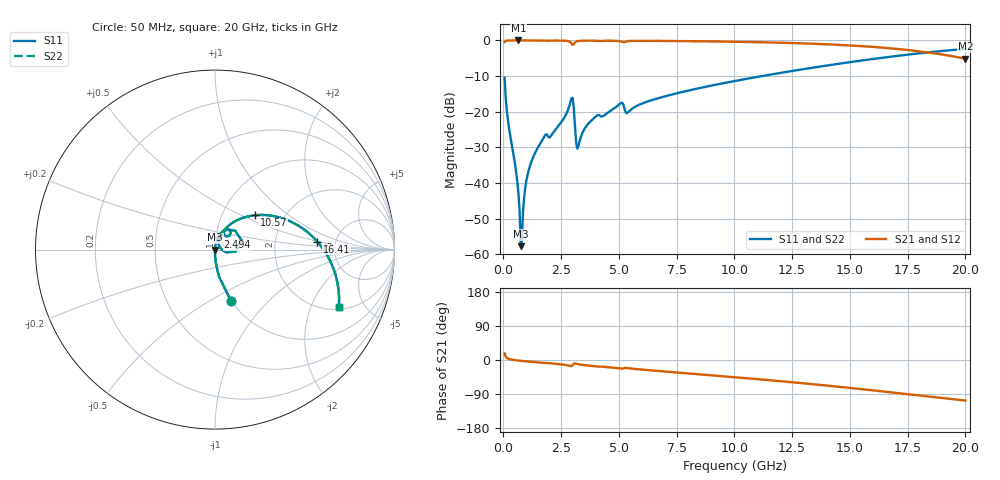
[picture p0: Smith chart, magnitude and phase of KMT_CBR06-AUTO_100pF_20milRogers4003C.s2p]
! Data measured by Modelithics Inc. support@modelithics.com 813-866-6335
! KEMET CBR06-AUTO 100pF, Pad Width= 0.851mm, Pad Length= 0.64mm, Pad Gap= 0.62mm, 20mil Rogers 4003C substrate Data, January 2022
# hz S ma R 50
! 2 Port Network Data from SP1.SP block
! freq  magS11  angS11  magS21  angS21  magS12  angS12  magS22  angS22
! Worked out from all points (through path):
!   401 points, 50 MHz to 20 GHz, reference 50 ohm
!   highest |S21| = 0.00 dB at 648.5 MHz (marker M1); lowest = -5.1 dB at 20 GHz (marker M2)
!   group delay of S21, straight-line fit = 14.9 ps
!   lowest |S11| = -57.7 dB at 748.2 MHz (marker M3), VSWR 1.00, Z = 50 - j0.125 ohm
!   |S11| at or under -10 dB: start of sweep to 11.18 GHz
!   |S22| runs from -57.7 to -2.4 dB; largest |S21 - S12| = 0
!   S11 on the Smith chart (normalised r, x): 50 MHz: 1.00, -0.63; 2.494 GHz: 1.03, +0.14; 10.57 GHz: 1.42, +0.59; 16.41 GHz: 3.61, +0.48; 20 GHz: 2.15, -3.23
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5e7  0.301 -72.6  0.9533 17.4  0.9533 17.4  0.301 -72.6
5.4875e8  0.01434 -89.3  0.9995 -0.8  0.9995 -0.8  0.01434 -89.3
6.485e8  0.007213 -88.3  0.9995 -1.5  0.9995 -1.5  0.007213 -88.3
7.4825e8  0.001304 -72.8  0.9995 -2.2  0.9995 -2.2  0.001304 -72.8
8.48e8  0.004034 80.6  0.9995 -2.8  0.9995 -2.8  0.004034 80.6
1.0475e9  0.0132 83.8  0.9993 -3.9  0.9993 -3.9  0.0132 83.8
1.296875e9  0.02351 83.2  0.999 -5.2  0.999 -5.2  0.02351 83.2
1.74575e9  0.04357 78.3  0.996 -7.7  0.996 -7.7  0.04357 78.3
2.493875e9  0.07067 75.8  0.994 -11.5  0.994 -11.5  0.07067 75.8
2.94275e9  0.154 42.9  0.9125 -16.4  0.9125 -16.4  0.154 42.9
3.192125e9  0.03043 25.1  0.975 -10.5  0.975 -10.5  0.03043 25.1
3.391625e9  0.04807 66.9  0.9902 -12.8  0.9902 -12.8  0.04807 66.9
3.990125e9  0.08544 69.0  0.9899 -16.8  0.9899 -16.8  0.08544 69.0
5.0375e9  0.1293 60.6  0.9758 -22.4  0.9758 -22.4  0.1293 60.6
5.386625e9  0.09758 58.0  0.9775 -21.5  0.9775 -21.5  0.09758 58.0
6.73325e9  0.156 60.0  0.9848 -29.0  0.9848 -29.0  0.156 60.0
1.0025e10  0.2703 43.8  0.9584 -45.3  0.9584 -45.3  0.2703 43.8
1.057362e10  0.2916 40.9  0.9516 -48.2  0.9516 -48.2  0.2916 40.9
1.336662e10  0.4137 24.9  0.9 -63.7  0.9 -63.7  0.4137 24.9
1.6409e10  0.5721 4.5  0.7927 -82.8  0.7927 -82.8  0.5721 4.5
1.670825e10  0.5886 2.2  0.778 -84.8  0.778 -84.8  0.5886 2.2
2e10  0.7599 -24.7  0.5547 -107.0  0.5547 -107.0  0.7599 -24.7
